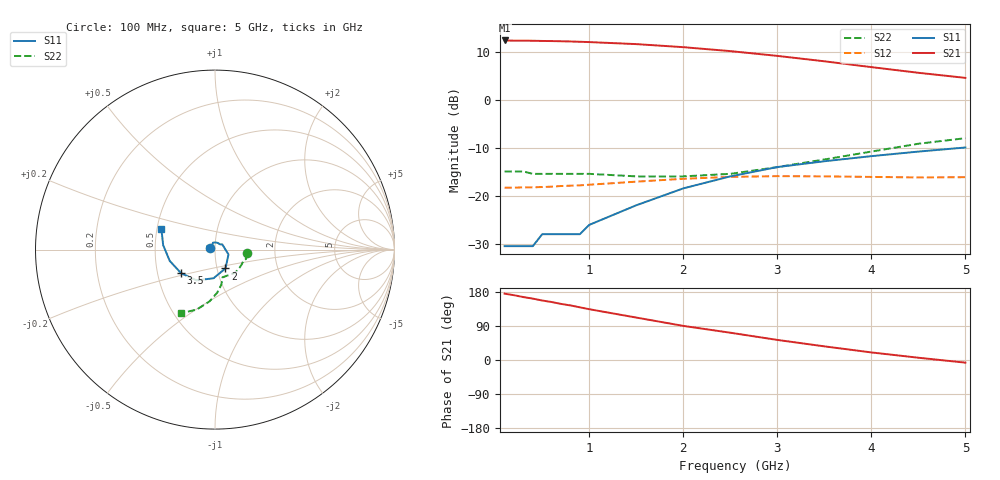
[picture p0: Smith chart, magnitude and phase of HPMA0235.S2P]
! HPMA-0235
! Typical S-Parameters, Z  = 50 , T  = 25 C, I  = 25mA
# ghz s ma r 50
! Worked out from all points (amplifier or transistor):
!   18 points, 100 MHz to 5 GHz, reference 50 ohm
!   highest |S21| = 12.4 dB at 100 MHz (marker M1)
!   |S21| within 3 dB of that: start of sweep to 2.892 GHz
!   unconditionally stable (mu >= 1): start of sweep to end of sweep
!   at 400 MHz: K = 1.21, MAG = 12.5 dB, |S12| = -18.2 dB
!   at 1 GHz: K = 1.19, MAG = 12.2 dB, |S12| = -17.7 dB
!   at 5 GHz: K = 1.46, MAG = 6.3 dB, |S12| = -16.1 dB
!   S11 on the Smith chart (normalised r, x): 100 MHz: 0.94, +0.01; 2 GHz: 1.10, -0.23; 3.5 GHz: 0.66, -0.18; 5 GHz: 0.53, +0.13
0.1  0.03 167.0  4.17 175.0  0.122 1.0  0.18 -6.0
0.2  0.03 151.0  4.15 171.0  0.122 2.0  0.18 -11.0
0.3  0.03 137.0  4.15 166.0  0.123 2.0  0.18 -17.0
0.4  0.03 122.0  4.14 162.0  0.123 3.0  0.17 -22.0
0.5  0.04 106.0  4.12 157.0  0.124 4.0  0.17 -27.0
0.6  0.04 91.0  4.11 153.0  0.125 5.0  0.17 -32.0
0.7  0.04 76.0  4.09 148.0  0.127 5.0  0.17 -36.0
0.8  0.04 62.0  4.07 144.0  0.128 6.0  0.17 -41.0
0.9  0.04 48.0  4.04 139.0  0.129 6.0  0.17 -46.0
1  0.05 35.0  4.01 134.0  0.131 7.0  0.17 -50.0
1.5  0.08 -20.0  3.82 112.0  0.141 7.0  0.16 -66.0
2  0.12 -61.0  3.55 90.0  0.151 6.0  0.16 -75.0
2.5  0.16 -93.0  3.23 72.0  0.158 5.0  0.17 -76.0
3  0.2 -121.0  2.88 53.0  0.161 2.0  0.2 -80.0
3.5  0.23 -145.0  2.53 36.0  0.16 -1.0  0.24 -87.0
4  0.26 -166.0  2.2 20.0  0.158 -2.0  0.29 -96.0
4.5  0.29 175.0  1.92 6.0  0.156 -2.0  0.35 -107.0
5  0.32 159.0  1.7 -7.0  0.157 -1.0  0.4 -118.0
